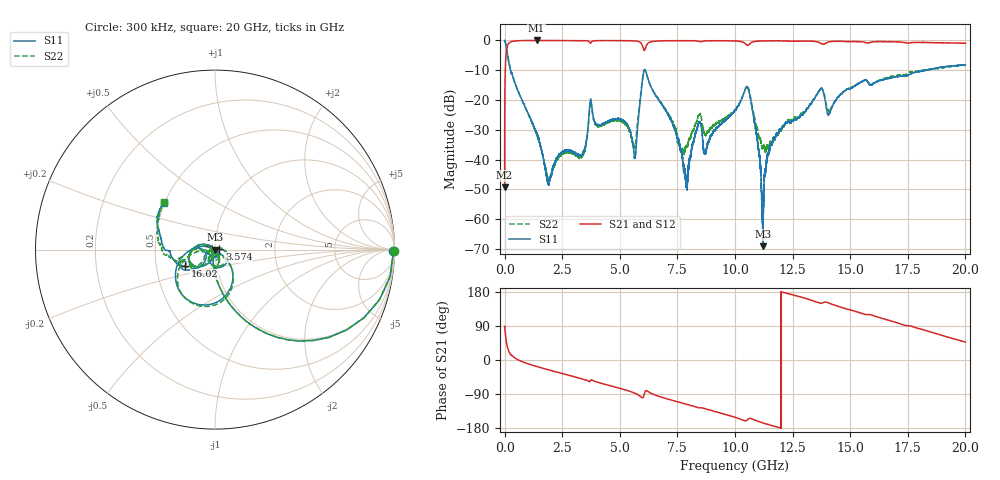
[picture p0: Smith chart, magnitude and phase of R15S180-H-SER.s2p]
!{R15S180}
!Johanson Technology Inc.
!www.johansontechnology.com
!Test Board Conditions:
!Substrate Type  RO4350B
!Substrate Thickness  20 mil
!Substrate Dk  3.66
!TL Type: GCPW
!TL Trace Width  34 mil
!TL Gap  10 mil
!Electrode orientation  Horizontal
!DUT TOPOLOGY	SERIES
!Mounting Pad LxW  26x52 mil
! Created Sat Feb  6 14:17:07 2021
# hz S ma R 50
! 2 Port Network Data from SP1.SP block
! freq  magS11  angS11  magS21  angS21  magS12  angS12  magS22  angS22
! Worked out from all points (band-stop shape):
!   20001 points, 300 kHz to 20 GHz, reference 50 ohm
!   highest |S21| = -0.01 dB at 1.388 GHz (marker M1); lowest = -49.3 dB at 300 kHz (marker M2)
!   |S21| within 3 dB of the highest: 88.46 MHz to 6.031 GHz (5.943 GHz wide, 194 % of centre); 6.094 GHz to end of sweep
!   lowest |S11| = -69.1 dB at 11.21 GHz (marker M3), VSWR 1.00, Z = 50 + j0.0105 ohm
!   |S11| at or under -10 dB: 259.9 MHz to 6.062 GHz (5.802 GHz wide, 184 % of centre); 6.102 GHz to 18.31 GHz (12.2 GHz wide, 100 % of centre)
!   |S22| runs from -47.3 to 0.0 dB; largest |S21 - S12| = 0.015
!   S11 on the Smith chart (normalised r, x): 300 kHz: open; 3.574 GHz: 1.05, +0.01; 16.02 GHz: 0.70, -0.13; 20 GHz: 0.50, +0.30
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300000  0.9944 -0.4  0.003432 88.6  0.003375 88.3  0.9955 -0.4
1.023e8  0.6501 -50.7  0.756 39.2  0.7568 39.1  0.6518 -50.6
1.633e8  0.4711 -63.8  0.8777 25.9  0.879 25.8  0.4727 -63.8
1.3883e9  0.02807 -111.2  0.9988 -17.0  0.9975 -17.0  0.02695 -102.5
1.9023e9  0.003864 157.9  0.9977 -25.8  0.9976 -25.8  0.004434 -37.8
3.3343e9  0.01159 23.8  0.995 -49.2  0.9954 -49.2  0.01093 47.1
3.5743e9  0.02434 7.9  0.989 -53.9  0.9893 -54.0  0.02202 29.4
3.7593e9  0.0941 -94.8  0.9289 -52.3  0.9283 -52.3  0.08735 -98.3
5.6403e9  0.01052 -117.5  0.9822 -87.2  0.9823 -87.2  0.0157 -95.9
6.0643e9  0.3169 -102.7  0.6773 -89.6  0.6798 -89.6  0.3231 -100.4
6.6673e9  0.1034 172.9  0.9798 -95.4  0.9794 -95.4  0.1054 -172.1
7.8833e9  0.004113 51.4  0.9904 -116.6  0.9902 -116.6  0.01697 -81.9
8.4223e9  0.04089 -62.0  0.9689 -126.0  0.9678 -126.0  0.0548 -70.0
8.7143e9  0.01278 -66.1  0.9828 -128.7  0.983 -128.7  0.02549 -80.9
1.00003e10  0.06671 -71.2  0.9806 -151.1  0.9797 -151.1  0.06831 -68.3
1.05873e10  0.1485 -165.3  0.8388 -155.0  0.8391 -155.1  0.1544 -162.2
1.12103e10  0.0003506 162.6  0.9825 -166.0  0.983 -165.9  0.01605 174.5
1.17353e10  0.02295 -68.1  0.9867 -175.3  0.9855 -175.3  0.02192 -126.6
1.33343e10  0.0909 -118.0  0.9705 157.3  0.9714 157.3  0.09045 -122.9
1.60223e10  0.1907 -151.9  0.9479 116.7  0.9488 116.9  0.1912 -161.0
1.66673e10  0.2309 -163.5  0.9536 104.8  0.9421 104.7  0.2428 -166.8
2e10  0.3844 137.7  0.8948 47.3  0.8891 47.0  0.3884 137.1
